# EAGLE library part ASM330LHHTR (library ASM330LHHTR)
STMICROELECTRONICS - ASM330LHHTR - MEMS MOD, 3-AXIS GYROSCOPE/ACCELEROMETER Source: Datasheet
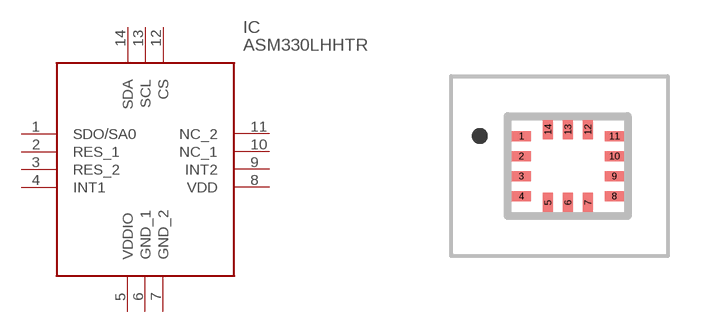
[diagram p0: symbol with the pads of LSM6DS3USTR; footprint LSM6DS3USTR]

Designator prefix IC

## ASM330LHHTR (Arrow_Part_Number: ASM330LHHTR; Arrow_Price-Stock: https://www.arrow.com/en/products/asm330lhhtr/stmicroelectronics?utm_currency=USD&region=europe; Description: STMICROELECTRONICS - ASM330LHHTR - MEMS MOD, 3-AXIS GYROSCOPE/ACCELEROMETER; Height: 0.86mm; Manufacturer_Name: STMicroelectronics; Manufacturer_Part_Number: ASM330LHHTR; Mouser_Part_Number: 511-ASM330LHHTR; Mouser_Price-Stock: https://www.mouser.co.uk/ProductDetail/STMicroelectronics/ASM330LHHTR?qs=lc2O%252BfHJPVYgP8P9MzExKQ%3D%3D)  [LSM6DS3USTR]
1  SDO/SA0
2  RES_1
3  RES_2
4  INT1
5  VDDIO
6  GND_1
7  GND_2
8  VDD
9  INT2
10  NC_1
11  NC_2
12  CS
13  SCL
14  SDA

## Footprint LSM6DS3USTR (pad centres in mm)
LGA-14(2.5x3x0.86)
smd 0.475 x 0.25: 1 -1.163,0.75; 2 -1.163,0.25; 3 -1.163,-0.25; 4 -1.163,-0.75; 8 1.163,-0.75; 9 1.163,-0.25; 10 1.163,0.25; 11 1.163,0.75
smd 0.25 x 0.475: 5 -0.5,-0.912; 6 0,-0.912; 7 0.5,-0.912; 12 0.5,0.912; 13 0,0.912; 14 -0.5,0.912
